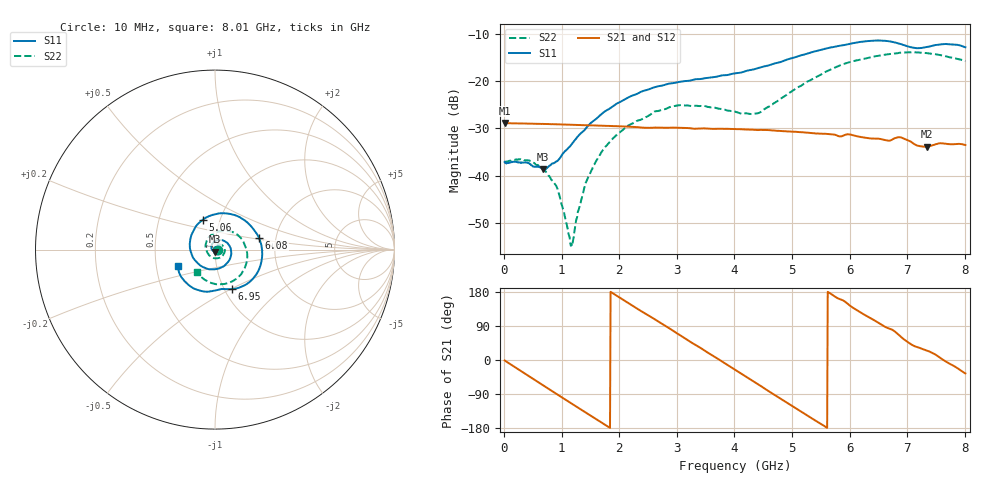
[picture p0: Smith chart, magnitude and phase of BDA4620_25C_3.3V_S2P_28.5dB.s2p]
!Agilent Technologies,E5071B,MY42404982,A.09.10
!Date: Wed May 06 08:55:01 2026
!Data & Calibration Information:
!Freq	S11:SOLT2(ON)	S21:SOLT2(ON)	S12:SOLT2(ON)	S22:SOLT2(ON)
# Hz S RI R 50
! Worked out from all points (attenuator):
!   801 points, 10 MHz to 8.01 GHz, reference 50 ohm
!   highest |S21| = -28.87 dB at 10 MHz (marker M1); lowest = -33.9 dB at 7.34 GHz (marker M2)
!   lowest |S11| = -38.7 dB at 680 MHz (marker M3), VSWR 1.02, Z = 49.8 - j1.14 ohm
!   |S11| at or under -10 dB: start of sweep to end of sweep
!   |S22| runs from -54.9 to -13.9 dB; largest |S21 - S12| = 0.00019
!   S11 on the Smith chart (normalised r, x): 10 MHz: 1.03, -0.00; 5.06 GHz: 0.83, +0.28; 6.08 GHz: 1.63, +0.23; 6.95 GHz: 1.08, -0.51; 8.01 GHz: 0.65, -0.13
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1e7  0.0139 -0.000866  0.036 -0.000763  0.036 -0.000784  0.014 -0.000468
4.2e8  0.00834 -0.0107  0.0265 -0.0235  0.0266 -0.0236  0.0136 -0.00491
6.8e8  -0.00185 -0.0115  0.0138 -0.0324  0.0138 -0.0324  0.0094 -0.00693
9.3e8  -0.0132 -0.00543  -0.000784 -0.0349  -0.000872 -0.035  0.00354 -0.00624
1.16e9  -0.0196 0.00727  -0.0138 -0.0316  -0.0139 -0.0317  -0.00141 -0.00114
1.2e9  -0.0202 0.00995  -0.016 -0.0305  -0.016 -0.0306  -0.00204 3.98e-05
1.35e9  -0.0199 0.0205  -0.023 -0.0254  -0.023 -0.0255  -0.00355 0.00456
1.53e9  -0.0143 0.0341  -0.0292 -0.0173  -0.0293 -0.0173  -0.00341 0.0112
1.77e9  0.00187 0.0484  -0.0333 -0.0044  -0.0333 -0.00441  0.000675 0.0205
2.14e9  0.0406 0.0523  -0.0292 0.0156  -0.0292 0.0156  0.0164 0.0291
2.68e9  0.0881 0.00439  -0.00628 0.0315  -0.00623 0.0315  0.0442 0.0196
3.08e9  0.0805 -0.0578  0.0145 0.0285  0.0145 0.0285  0.0552 -0.00715
4.01e9  -0.0826 -0.0879  0.028 -0.0136  0.028 -0.0136  -0.0102 -0.0465
4.42e9  -0.1379 -0.00122  0.0128 -0.0275  0.0128 -0.0276  -0.0443 -0.0128
5.06e9  -0.0693 0.1652  -0.0175 -0.0233  -0.0175 -0.0233  -0.0238 0.0794
5.35e9  0.0215 0.2015  -0.0254 -0.0121  -0.0255 -0.0121  0.023 0.1017
6.08e9  0.2442 0.0669  -0.019 0.0185  -0.019 0.0186  0.1569 0.0461
6.68e9  0.1926 -0.1804  0.00267 0.0232  0.0027 0.0233  0.1702 -0.09
6.95e9  0.0942 -0.22  0.0145 0.0198  0.0146 0.0199  0.1351 -0.1482
7.34e9  -0.00305 -0.2286  0.0183 0.00843  0.0184 0.00851  0.0431 -0.1928
7.66e9  -0.1211 -0.2152  0.0217 -0.00115  0.0218 -0.00112  -0.0349 -0.1802
8.01e9  -0.2082 -0.0927  0.0171 -0.0122  0.0171 -0.0122  -0.1017 -0.1275
